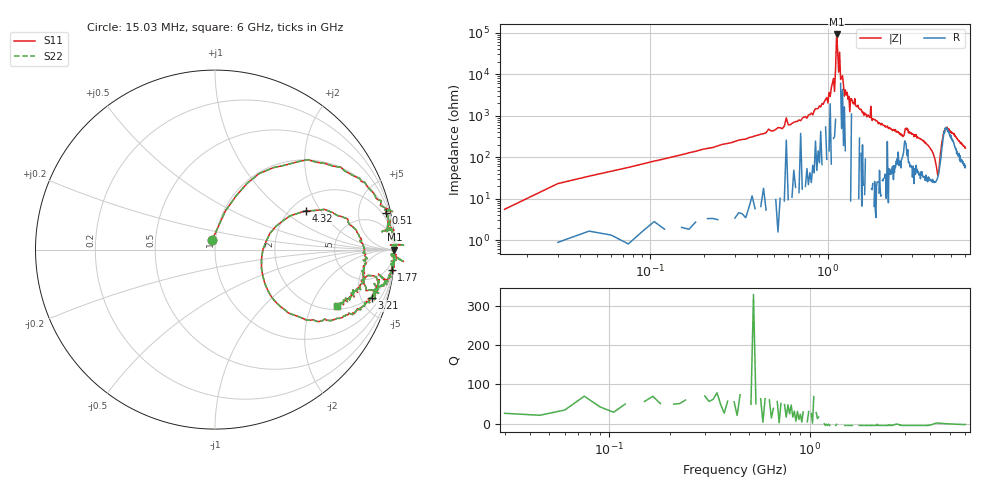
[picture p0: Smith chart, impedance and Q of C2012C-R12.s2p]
!	Network	Analyzer	HP8753E.07.74:	Oct	30	2002	Serial	No.	JP38451487
!	Hewlett-Packard
!	7	Sep	2009	12:14:06
!	Frequency	S11	S21	S12	S22
#	HZ	S	RI	R	50
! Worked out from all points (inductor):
!   400 points, 15.03 MHz to 6 GHz, reference 50 ohm
!   read as one part in series: L = 121 nH near 45.03 MHz
!   highest |Z| = 91.2 kohm at 1.125 GHz (marker M1)
!   self-resonance near 1.11 GHz
!   S11 on the Smith chart (normalised r, x): 15.03 MHz: 0.96, +0.10; 510 MHz: 1.21, +9.33; 1.77 GHz: 1, -17; 3.21 GHz: 1.87, -6.05; 4.32 GHz: 2.39, +1.48; 6 GHz: 2.18, -3.11
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1.502992e7  -0.0154 0.0536  1.02 -0.0536  1.02 -0.0536  -0.0154 0.0536
3.002985e7  0.0576 0.215  0.942 -0.215  0.942 -0.215  0.0576 0.215
1.050295e8  0.396 0.472  0.604 -0.472  0.604 -0.472  0.396 0.472
5.100274e8  0.952 0.203  0.0476 -0.203  0.0476 -0.203  0.952 0.203
1.020025e9  0.998 0.0272  0.0018 -0.0272  0.0018 -0.0272  0.998 0.0272
1.095025e9  0.997 0.0256  0.00272 -0.0256  0.00272 -0.0256  0.997 0.0256
1.125024e9  1 -0.000122  -0.00109 0.000122  -0.00109 0.000122  1 -0.000122
1.155024e9  1 0.00842  -0.0028 -0.00842  -0.0028 -0.00842  1 0.00842
1.170024e9  1 -0.00287  -0.00067 0.00287  -0.00067 0.00287  1 -0.00287
1.185024e9  0.989 -0.00772  0.0108 0.00772  0.0108 0.00772  0.989 -0.00772
1.335023e9  1.05 -0.0663  -0.0522 0.0663  -0.0522 0.0663  1.05 -0.0663
1.425023e9  1 -0.0388  -0.00128 0.0388  -0.00128 0.0388  1 -0.0388
1.770021e9  0.985 -0.114  0.0155 0.114  0.0155 0.114  0.985 -0.114
2.01002e9  0.973 -0.153  0.027 0.153  0.027 0.153  0.973 -0.153
3.015015e9  0.912 -0.242  0.0882 0.242  0.0882 0.242  0.912 -0.242
3.210014e9  0.872 -0.27  0.128 0.27  0.128 0.27  0.872 -0.27
4.00501e9  0.506 -0.391  0.494 0.391  0.494 0.391  0.506 -0.391
4.200009e9  0.259 -0.0533  0.741 0.0533  0.741 0.0533  0.259 -0.0533
4.320008e9  0.505 0.216  0.495 -0.216  0.495 -0.216  0.505 0.216
4.605007e9  0.832 0.00531  0.168 -0.00531  0.168 -0.00531  0.832 0.00531
5.010005e9  0.827 -0.119  0.173 0.119  0.173 0.119  0.827 -0.119
6e9  0.679 -0.314  0.321 0.314  0.321 0.314  0.679 -0.314
